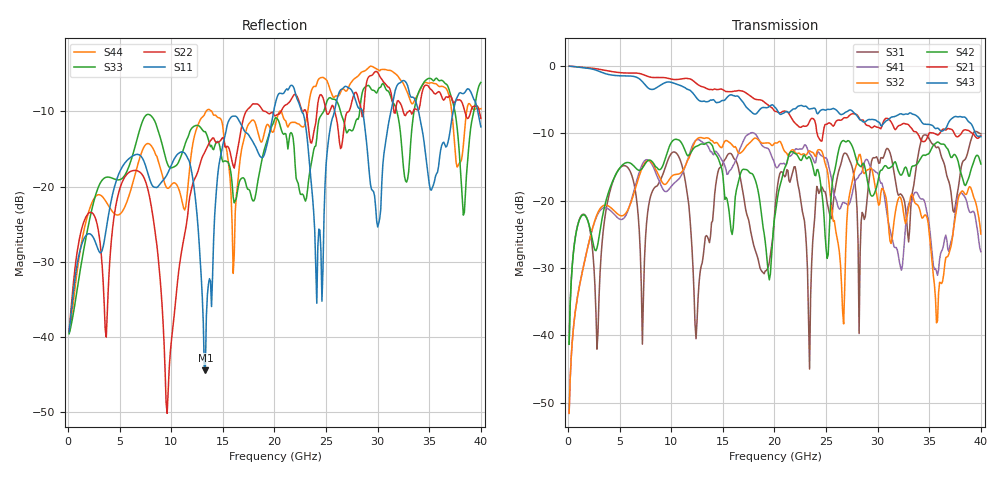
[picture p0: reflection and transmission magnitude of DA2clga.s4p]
! ADC12DJ3200QML-SP
! 196-pin ZMX package
! CLGA Ceramic Package without columns (ceramic land grid array)
! Texas Instruments 4/21/2021
! Single-ended  S-parameters
! PORT#  PORT_NAME  NET_NAME
! PORT1:  DAxN.DIEBUMP DAxN
! PORT2:  DAxN.BGA  DAxN
! PORT3:  DAxP.DIEBUMP DAxP
! PORT4:  DAxP.BGA  DAxP
! Touchstone Ver. 1.0
! Number of ports is 4
# Hz	S	MA	R	50.000000
! SCATTERING PARAMETERS  :
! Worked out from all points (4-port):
!   400 points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, 100 MHz to 40 GHz, reference 50 ohm
!   strongest paths, dB at 100 MHz, 10.1 GHz, 20.1 GHz, 30.1 GHz, 40 GHz:
!     S43: -0.1, -2.5, -6.3, -8.4, -10.6
!     S21: -0.1, -2.0, -6.8, -9.2, -10.4
!     S42: -41.3, -11.2, -21.7, -16.5, -14.6
!     S32: -51.5, -16.3, -11.5, -20.7, -25.0
!     S41: -51.5, -17.7, -14.9, -16.3, -27.6
!     S31: -41.3, -12.9, -20.4, -14.5, -10.1
!   lowest |S11| = -44.5 dB at 13.3 GHz (marker M1), VSWR 1.01, Z = 49.6 - j0.439 ohm
!   |S11| at or under -10 dB: start of sweep to 19.92 GHz; 22.64 GHz to 25.81 GHz (3.17 GHz wide, 13.1 % of centre); 33.96 GHz to 37.32 GHz (3.367 GHz wide, 9.45 % of centre)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
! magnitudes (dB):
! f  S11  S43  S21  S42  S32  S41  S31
! 100 MHz  -39.4  -0.1  -0.1  -41.3  -51.5  -51.5  -41.3
! 11.1 GHz  -15.4  -3.1  -1.9  -11.8  -15.6  -15.9  -15.2
! 13.3 GHz  -44.5  -5.3  -3.3  -11.6  -10.7  -11.5  -25.4
! 15.8 GHz  -10.8  -4.3  -3.9  -24.5  -11.6  -15.4  -13.1
! 23.4 GHz  -17.1  -6.4  -8.3  -13.6  -12.6  -13.0  -45.0
! 24.1 GHz  -35.5  -7.1  -9.9  -15.5  -12.8  -13.2  -17.9
! 40 GHz  -12.1  -10.6  -10.4  -14.6  -25.0  -27.6  -10.1
